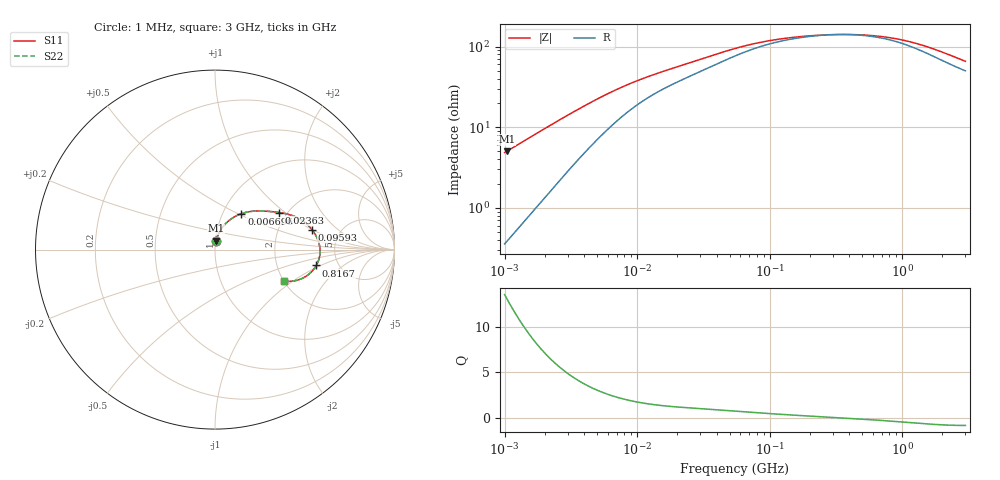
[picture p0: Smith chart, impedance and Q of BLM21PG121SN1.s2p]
! BLM21PG121SN1
# Hz S RI R 50
!Freq.(Hz) S11(Real) S11(Imag) S21(Real) S21(Imag) S12(Real) S12(Imag) S22(Real) S22(Imag)
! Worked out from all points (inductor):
!   401 points, 1 MHz to 3 GHz, reference 50 ohm
!   read as one part in series: L = 766 nH near 1.041 MHz
!   highest Q = 13.1 at 1.041 MHz (marker M1), where L = 769 nH
!   self-resonance near 334.4 MHz
!   S11 on the Smith chart (normalised r, x): 1 MHz: 1.01, +0.10; 6.696 MHz: 1.22, +0.52; 23.63 MHz: 1.82, +0.91; 95.93 MHz: 3.12, +1.00; 816.7 MHz: 3.41, -0.89; 3 GHz: 2.00, -0.85
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1000000  0.00586 0.0479  0.9941 -0.0479  0.9941 -0.0479  0.00586 0.0479
1040844  0.00632 0.0498  0.9937 -0.0498  0.9937 -0.0498  0.00632 0.0498
2182827  0.0255 0.0989  0.9745 -0.0989  0.9745 -0.0989  0.0255 0.0989
3823119  0.0674 0.1527  0.9326 -0.1527  0.9326 -0.1527  0.0674 0.1527
5059610  0.1027 0.1793  0.8973 -0.1793  0.8973 -0.1793  0.1027 0.1793
6696013  0.147 0.2002  0.853 -0.2002  0.853 -0.2002  0.147 0.2002
9600343  0.2106 0.2138  0.7894 -0.2138  0.7894 -0.2138  0.2106 0.2138
1.461624e7  0.2821 0.2143  0.7179 -0.2143  0.7179 -0.2143  0.2821 0.2143
2.362996e7  0.3577 0.2066  0.6423 -0.2066  0.6423 -0.2066  0.3577 0.2066
3.670325e7  0.4271 0.1909  0.5729 -0.1909  0.5729 -0.1909  0.4271 0.1909
5.477226e7  0.4848 0.1633  0.5152 -0.1633  0.5152 -0.1633  0.4848 0.1633
9.593103e7  0.5412 0.1108  0.4588 -0.1108  0.4588 -0.1108  0.5412 0.1108
1.403209e8  0.5635 0.0755  0.4365 -0.0755  0.4365 -0.0755  0.5635 0.0755
2.094008e8  0.5778 0.0406  0.4222 -0.0406  0.4222 -0.0406  0.5778 0.0406
4.304467e8  0.5848 -0.0231  0.4152 0.0231  0.4152 0.0231  0.5848 -0.0231
5.929311e8  0.5787 -0.0544  0.4213 0.0544  0.4213 0.0544  0.5787 -0.0544
8.005644e8  0.5654 -0.0861  0.4346 0.0861  0.4346 0.0861  0.5654 -0.0861
8.167498e8  0.5642 -0.0883  0.4358 0.0883  0.4358 0.0883  0.5642 -0.0883
1.147801e9  0.5361 -0.1253  0.4639 0.1253  0.4639 0.1253  0.5361 -0.1253
1.581072e9  0.495 -0.156  0.505 0.156  0.505 0.156  0.495 -0.156
2.177892e9  0.4412 -0.1745  0.5588 0.1745  0.5588 0.1745  0.4412 -0.1745
3e9  0.383 -0.1747  0.617 0.1747  0.617 0.1747  0.383 -0.1747
